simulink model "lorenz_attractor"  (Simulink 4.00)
settings: Solver=ode23  SolverMode=SingleTasking  StartTime=0.0  StopTime=100  FixedStep=0.01  RelTol=1e-3
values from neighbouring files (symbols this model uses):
  beta = 1    [lorenz_attractor_ini.m]
  rho = 26.5    [lorenz_attractor_ini.m]
  sigma = 3    [lorenz_attractor_ini.m]
libraries: simulink3 x1

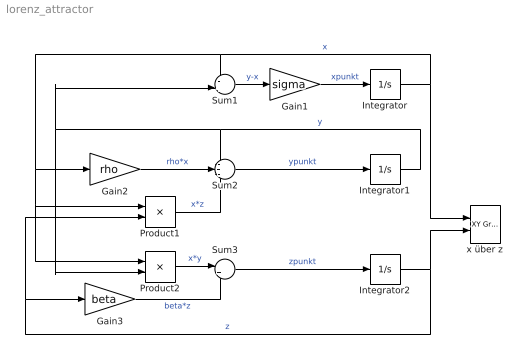
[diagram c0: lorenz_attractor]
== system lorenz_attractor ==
  Gain1 : Gain  Gain=sigma  Multiplication=Element-wise(K.*u)  SaturateOnIntegerOverflow=on
  Gain2 : Gain  Gain=rho  Multiplication=Element-wise(K.*u)  SaturateOnIntegerOverflow=on
  Gain3 : Gain  Gain=beta  Multiplication=Element-wise(K.*u)  SaturateOnIntegerOverflow=on
  Integrator : Integrator  ExternalReset=none  InitialConditionSource=internal  InitialCondition=5  LimitOutput=off  UpperSaturationLimit=inf  LowerSaturationLimit=-inf  ShowSaturationPort=off  ShowStatePort=off  AbsoluteTolerance=auto
  Integrator1 : Integrator  ExternalReset=none  InitialConditionSource=internal  InitialCondition=5  LimitOutput=off  UpperSaturationLimit=inf  LowerSaturationLimit=-inf  ShowSaturationPort=off  ShowStatePort=off  AbsoluteTolerance=auto
  Integrator2 : Integrator  ExternalReset=none  InitialConditionSource=internal  InitialCondition=5  LimitOutput=off  UpperSaturationLimit=inf  LowerSaturationLimit=-inf  ShowSaturationPort=off  ShowStatePort=off  AbsoluteTolerance=auto
  Product1 : Product  Inputs=2  Multiplication=Element-wise(.*)  SaturateOnIntegerOverflow=on
  Product2 : Product  Inputs=2  Multiplication=Element-wise(.*)  SaturateOnIntegerOverflow=on
  Sum1 : Sum  Inputs=-+|  SaturateOnIntegerOverflow=on
  Sum2 : Sum  Inputs=-+-  SaturateOnIntegerOverflow=on
  Sum3 : Sum  Inputs=|+-  SaturateOnIntegerOverflow=on
  x über z : simulink3/Sinks/XY Graph  xmin=-15  xmax=15  ymin=0  ymax=50  st=-1
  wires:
  Sum1/1 -> Gain1/1  "y-x"
  Gain1/1 -> Integrator/1  "xpunkt"
  Integrator/1 -> x über z/1, Sum1/1, Gain2/1, Product1/1, Product2/1  "x"
  Integrator2/1 -> x über z/2, Product1/2, Gain3/1  "z"
  Product1/1 -> Sum2/3  "x*z"
  Sum2/1 -> Integrator1/1  "ypunkt"
  Gain2/1 -> Sum2/2  "rho*x"
  Product2/1 -> Sum3/1  "x*y"
  Gain3/1 -> Sum3/2  "beta*z"
  Integrator1/1 -> Sum2/1, Product2/2, Sum1/2  "y"
  Sum3/1 -> Integrator2/1  "zpunkt"
